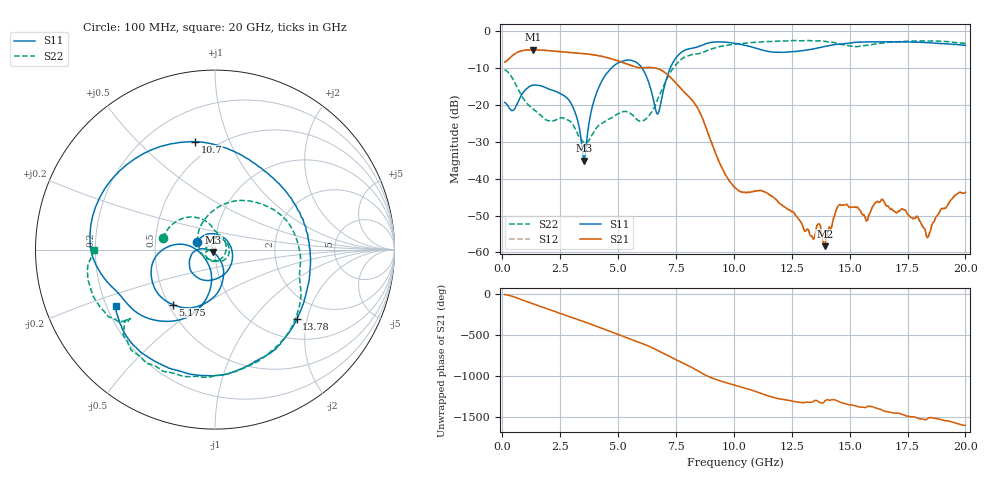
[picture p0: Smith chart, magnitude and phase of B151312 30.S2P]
!  2-Port S-parameters saved by WinCal
! VAR MeasName=S-Parameters (CALIBRATED_DATA) read from VNA (N5244A)
! VAR MeasDate=12/8/2015 5:45:47 PM
! VAR NAME=B151312 30
! VAR FILENAME=B151312 30.S2P
! VAR DATE=12/8/2015 5:45:47 PM
! VAR PHYS_PORTS=1,2
# Hz S DB R 50
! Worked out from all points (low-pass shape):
!   401 points, 100 MHz to 20 GHz, reference 50 ohm
!   highest |S21| = -5.15 dB at 1.344 GHz (marker M1); lowest = -58.3 dB at 13.93 GHz (marker M2)
!   |S21| within 3 dB of the highest: 188.9 MHz to 4.995 GHz (4.806 GHz wide, 185 % of centre)
!   lowest |S11| = -35.1 dB at 3.533 GHz (marker M3), VSWR 1.04, Z = 49 - j1.41 ohm
!   |S11| at or under -10 dB: start of sweep to 4.73 GHz; 6.026 GHz to 7.26 GHz (1.234 GHz wide, 18.6 % of centre)
!   |S22| runs from -30.4 to -2.6 dB; largest |S21 - S12| = 0.0014
!   S11 on the Smith chart (normalised r, x): 100 MHz: 0.82, +0.07; 5.175 GHz: 0.53, -0.38; 10.7 GHz: 0.39, +0.75; 13.78 GHz: 1.43, -1.73; 20 GHz: 0.24, -0.25
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1e8  -19.41 157.3  -8.48 -4.7  -8.48 -4.7  -10.57 167.6
6.4725e8  -19.73 -18.0  -5.86 -47.8  -5.86 -47.7  -15.36 109.0
1.34375e9  -14.72 -116.8  -5.15 -120.0  -5.15 -120.0  -21.23 72.5
1.94075e9  -15.60 -149.1  -5.35 -179.3  -5.36 -179.3  -24.21 -4.7
2.5875e9  -17.30 -166.6  -5.73 117.5  -5.73 117.5  -23.60 -112.2
3.43325e9  -30.86 -171.5  -6.16 33.5  -6.16 33.5  -29.57 -178.8
3.53275e9  -35.14 -124.6  -6.21 23.3  -6.21 23.3  -30.14 -172.8
4.42825e9  -12.25 -87.2  -7.12 -71.3  -7.12 -71.4  -24.64 125.1
5.1745e9  -8.27 -127.5  -8.55 -151.9  -8.53 -151.9  -22.02 -2.1
6.11975e9  -10.96 179.0  -10.01 108.1  -10.02 108.0  -24.21 -111.0
6.7665e9  -21.80 -122.8  -10.39 23.2  -10.40 23.2  -17.72 136.0
7.71175e9  -5.96 -127.9  -15.65 -110.4  -15.59 -110.5  -7.83 30.5
9.00525e9  -3.17 178.6  -29.79 59.4  -29.78 58.7  -5.00 -32.8
1.005e10  -3.42 131.2  -42.45 -35.5  -42.47 -35.7  -3.65 -65.0
1.069675e10  -4.27 100.5  -43.71 -88.5  -43.73 -88.9  -3.25 -79.9
1.338325e10  -4.99 -25.6  -55.60 118.5  -55.62 120.5  -2.74 -124.1
1.378125e10  -4.47 -40.5  -54.35 107.5  -54.12 106.7  -2.75 -130.1
1.39305e10  -4.26 -45.1  -58.29 133.5  -57.59 132.4  -2.90 -131.9
1.457725e10  -3.65 -67.0  -47.02 118.7  -47.03 119.9  -3.61 -140.1
1.67165e10  -3.02 -113.7  -47.92 -5.2  -47.69 -5.2  -3.11 -147.6
1.8408e10  -3.24 -137.0  -55.60 -75.5  -55.45 -78.7  -2.78 -164.5
2e10  -3.96 -150.3  -43.73 -167.2  -43.73 -168.0  -3.43 -179.6
